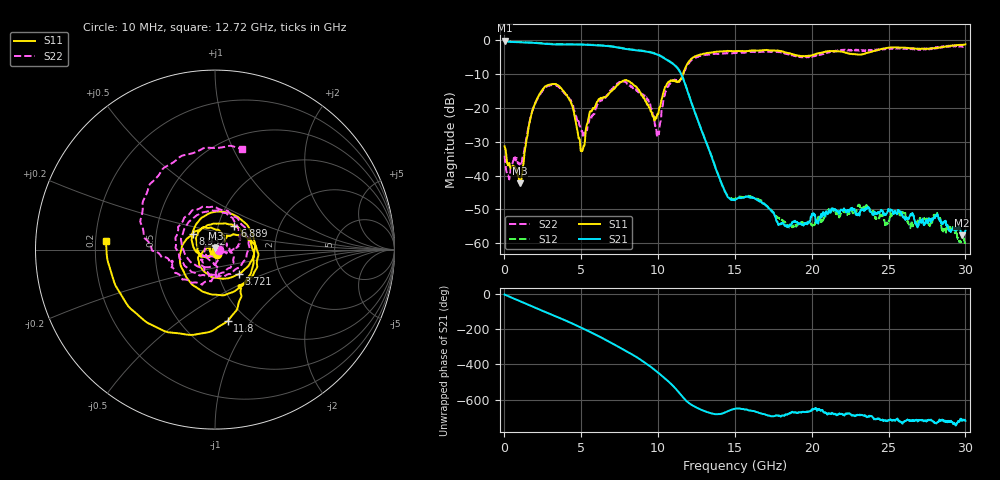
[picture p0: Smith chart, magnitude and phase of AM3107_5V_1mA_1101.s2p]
# Hz S DB R 50.0
!freq dBS11 angS11 dBS21 angS21 dBS12 angS12 dBS22 angS22
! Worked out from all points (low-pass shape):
!   1601 points, 10 MHz to 30 GHz, reference 50 ohm
!   highest |S21| = -0.19 dB at 10 MHz (marker M1); lowest = -57.7 dB at 29.76 GHz (marker M2)
!   |S21| within 3 dB of the highest: start of sweep to 8.956 GHz
!   lowest |S11| = -42.2 dB at 1.003 GHz (marker M3), VSWR 1.02, Z = 50.3 + j0.731 ohm
!   |S11| at or under -10 dB: start of sweep to 11.62 GHz
!   |S22| runs from -41.1 to -1.5 dB; largest |S21 - S12| = 0.013
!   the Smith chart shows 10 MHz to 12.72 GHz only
!   S11 on the Smith chart (normalised r, x): 10 MHz: 1.02, -0.05; 3.721 GHz: 1.26, -0.35; 6.889 GHz: 1.19, +0.32; 8.932 GHz: 0.77, +0.14; 11.8 GHz: 0.82, -0.78; 12.72 GHz: 0.24, +0.04
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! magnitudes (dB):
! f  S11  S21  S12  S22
! 10 MHz  -31.4  -0.2  -0.1  -34.1
! 1.003 GHz  -42.2  -0.6  -0.6  -36.6
! 2.109 GHz  -17.4  -0.9  -0.8  -17.6
! 3.721 GHz  -14.4  -1.3  -1.2  -14.6
! 4.377 GHz  -19.1  -1.3  -1.2  -18.5
! 5.015 GHz  -32.7  -1.3  -1.2  -26.8
! 5.633 GHz  -21.0  -1.4  -1.3  -23.2
! 6.889 GHz  -15.4  -1.8  -1.7  -14.9
! 8.932 GHz  -16.3  -3.2  -3.1  -16.2
! 10.02 GHz  -21.6  -4.4  -4.3  -27.6
! 10.6 GHz  -12.8  -5.9  -5.8  -13.7
! 11.8 GHz  -7.9  -13.5  -13.4  -8.3
! 12.72 GHz  -4.3  -25.3  -25.2  -4.7
! 14.29 GHz  -3.2  -44.1  -44.3  -3.9
! 15.01 GHz  -3.2  -47.3  -46.8  -3.8
! 18.36 GHz  -3.7  -54.9  -54.4  -4.1
! 20.01 GHz  -4.5  -51.4  -54.7  -4.9
! 23.12 GHz  -4.3  -51.1  -48.6  -2.9
! 25.01 GHz  -2.2  -50.1  -53.6  -2.6
! 28.09 GHz  -2.3  -51.9  -51.9  -2.1
! 29.76 GHz  -1.4  -57.7  -58.8  -1.7
! 30 GHz  -1.3  -56.2  -60.8  -1.6
